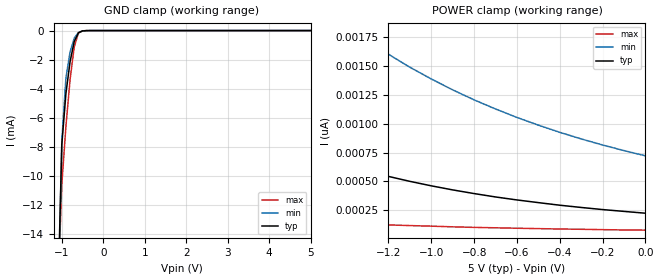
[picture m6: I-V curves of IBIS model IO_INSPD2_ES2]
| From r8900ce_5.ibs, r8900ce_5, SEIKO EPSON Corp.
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[Model]   IO_INSPD2_ES2
Model_type Input
Enable Active-Low
Polarity Non-Inverting
Vinh=4.0
Vinl=1.0
C_comp   2.5p   2p   3p
[Temperature Range] 25   85   -40
[Voltage Range]   5.0   4.5   5.5
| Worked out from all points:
|   GND clamp passes 1 mA (typ) near -0.72 V on its own axis
[GND Clamp]
-5V       -764.7mA   -643.6mA   -958.7mA
-1.1V     -19.19mA   -20.8mA    -18.4mA
-1V       -7.857mA   -7.617mA   -10.6mA
-900mV    -4.309mA   -3.241mA   -6.564mA
-800mV    -2.131mA   -1.46mA    -3.357mA
-700mV    -747.4uA   -523.1uA   -1.119mA
-600mV    -155uA     -130.4uA   -169.7uA
-500mV    -23.23uA   -25.44uA   -15.75uA
-400mV    -3.177uA   -4.273uA   -1.427uA
5V        224.8pA    987.9pA    66.96pA
[POWER Clamp]
-5V       19.86nA    40.44nA    3.589nA
-4.4V     11.28nA    24.06nA    1.932nA
-4.3V     10.25nA    22.04nA    1.741nA
-3.9V     6.969nA    15.49nA    1.153nA
-3.5V     4.718nA    10.87nA    767.4pA
-3V       2.89nA     6.993nA    470.9pA
-2.5V     1.776nA    4.533nA    299.5pA
-2.3V     1.465nA    3.825nA    254.2pA
-2V       1.105nA    2.983nA    201.2pA
-1.4V     645.3pA    1.86nA     136.7pA
-700mV    365.6pA    1.128nA    98.23pA
0V        224.8pA    722.1pA    77.99pA
